[IBIS Ver]   4.1
[File Name]   tms570ls31x_21x_revb_pge_a.ibs
[File Rev]   1.0
[Date]   Tue Sep 17 07:21:23 2013
[Source]   Texas Instruments, Inc.
[Notes]   Revision History:
   1.0: initial release, 09/17/2013
   THIS IS RELEASE 1.0,THE CONTENTS ARE SUBJECT TO
   CHANGE WITHOUT PRIOR NOTICE,IF NECESSARY.
[Disclaimer] Please be aware that in the absence of a written agreement
   Texas Instruments(TI) assumes no liability for:
   (1) The accuracy of the IBIS models provided to your company
   (2) The proper functioning of these Models in your design
   or for any resulting applications;or
   (3) Infringement of patents,copyrights or intellectual
   property rights resulting from your use of these models.
   TI provides IBIS Models as a service to our customers and
   therefore reserves the right to limit distribution of the
   Models.
[Copyright]   Property of Texas Instruments Incorporated.
   Unauthorised reproduction and/or distribution is strictly.
   prohibited.
   This product is protected under copyright law and trade
   secret law as an unpublished work.
   Created 2013,(C) Copyright 2013-2014,
   Texas Instruments Incorporated., All Rights Reserved.
   These commodities are under the U.S. Government
   distribution license control.As such,they are not to be
   re-exported without the prior approval of the
   U.S. Department of Commerce.
[Component]   TMS570LS31x/21x_REVB_PGE_A
[Manufacturer]   Texas Instruments
[Package]
| variable   typ   min   max
R_pkg   203.864m   14.6492m   240.64m
L_pkg   7.02358nH   2.16743nH   7.77511nH
C_pkg   0.954257pF   0.768716pF   6.71726pF
[Pin]	signal_name	model_name	R_pin	L_pin	C_pin
1	GIOB[3]	BQ0210FT	222.975m	6.99501nH	0.93522pF
2	GIOA[0]	BQ0210FT	224.24m	7.38373nH	1.04917pF
3	MIBSPI3NCS[3]	BQ0210FT	223.892m	7.5187nH	1.04438pF
4	MIBSPI3NCS[2]	BQ0210FT	218.592m	7.59933nH	1.02569pF
5	GIOA[1]	BQ0210FT	218.18m	7.74551nH	1.00793pF
6	NHET1[11]	BQ0210FT	219.431m	7.77511nH	0.979037pF
|7	FLTP1	BAFTHRU15VFT	219.36m	7.69214nH	0.954057pF
|8	FLTP2	BAFTHRU8VFT	219.133m	7.68768nH	0.936523pF
9	GIOA[2]	BQ0215FT	222.776m	7.74151nH	0.909504pF
|10	VCCIO	VDDS33TF1_60UM	225.672m	7.66706nH	0.910106pF
|11	VSS	VSS00T2_60UM	224.592m	7.55399nH	0.899234pF
12	CAN3RX	BQ0210FT	225.127m	7.44625nH	0.865528pF
13	CAN3TX	BQ0210FT	233.703m	7.53614nH	0.859082pF
14	GIOA[5]	BQ0210FT	233.974m	7.45808nH	0.855654pF
15	NHET1[22]	BQ0215FT	234.031m	7.40297nH	0.854333pF
16	GIOA[6]	BQ0210FT	233.473m	7.31284nH	0.840194pF
|17	VCC	VDD12T1_100UM	143.652m	6.76561nH	0.863346pF
|18	OSCIN	IOSCHF33FTHY_NI	236.172m	7.35407nH	0.808573pF
|19	KELVIN_GND	VSS00T2_60UM	234.204m	7.32997nH	0.824803pF
|20	OSCOUT	OOSCHF33FT	230.471m	7.21233nH	0.834372pF
|21	VSS	VSS00T2_60UM	230.586m	7.16874nH	0.824864pF
22	GIOA[7]	BQ0210FT	229.213m	7.20298nH	0.824815pF
23	NHET1[01]	BQ0215FT	228.006m	7.16514nH	0.860924pF
24	NHET1[03]	BQ0215FT	227.34m	7.17463nH	0.878282pF
25	NHET1[0]	BQ0215FT	228.05m	7.17956nH	0.888602pF
|26	VCCIO	VDDS33TF1_60UM	142.679m	6.74705nH	0.965478pF
|27	VSS	VSS00T2_60UM	226.431m	7.1827nH	0.927108pF
|28	VSS	VSS00T2_60UM	226.676m	7.26977nH	0.947242pF
|29	VCC	VDD12T1_100UM	144.773m	6.89389nH	1.01996pF
30	NHET1[02]	BQ0215FT	224.882m	7.39158nH	0.965642pF
31	NHET1[05]	BQ0215FT	224.815m	7.46872nH	0.970215pF
32	MIBSPI5NCS[0]	BQ0210FT	224.229m	7.54786nH	1.00261pF
33	NHET1[07]	BQ0215FT	225.045m	7.61055nH	1.02855pF
34	TEST	BQ0213FT	230.338m	7.61528nH	1.04296pF
35	NHET1[09]	BQ0215FT	226.956m	7.38938nH	1.04678pF
36	NHET1[04]	BQ0210FT	224.889m	7.05005nH	0.930999pF
37	MIBSPI3NCS[1]	BQ0215FT	212.649m	6.95179nH	0.940286pF
38	NHET1[06]	BQ0210FT	209.151m	7.19337nH	1.05396pF
39	NHET1[13]	BQ0210FT	211.994m	7.38781nH	1.03563pF
40	MIBSPI1NCS[2]	BQ0215FT	203.865m	7.31168nH	1.02434pF
41	NHET1[15]	BQ0210FT	197.232m	7.17257nH	0.997865pF
|42	VCCIO	VDDS33TF1_60UM	193.515m	7.14097nH	0.960455pF
|43	VSS	VSS00T2_60UM	189.265m	7.01956nH	0.944505pF
|44	VSS	VSS00T2_60UM	187.979m	6.89986nH	0.934945pF
|45	VCC	VDD12T1_100UM	101.964m	6.14255nH	0.970118pF
46	nPORRST	IQ0087FT	188.154m	6.76798nH	0.87611pF
|47	VSS	VSS00T2_60UM	189.169m	6.716nH	0.871341pF
|48	VCC	VDD12T1_100UM	124.671m	6.12514nH	0.899774pF
|49	VCC	VDD12T1_100UM	124.517m	6.02737nH	0.884127pF
|50	VSS	VSS00T2_60UM	192.682m	6.41208nH	0.826834pF
51	MIBSPI3SOMI	BQ0211FT	190.675m	6.39926nH	0.804598pF
52	MIBSPI3SIMO	BQ0211FT	189.543m	6.38502nH	0.794641pF
53	MIBSPI3CLK	BQ0211FT	191.031m	6.44993nH	0.78565pF
54	MIBSPI3NENA	BQ0210FT	193.5m	6.48248nH	0.784395pF
55	MIBSPI3NCS[0]	BQ0210FT	196.751m	6.3841nH	0.784861pF
|56	VSS	VSS00T2_60UM	197.376m	6.37405nH	0.784546pF
|57	VCC	VDD12T1_100UM	99.2024m	5.75114nH	0.844285pF
|58	AD1IN[16]_AD2IN[0]	IQ0444FT5	187.646m	6.39966nH	0.792979pF
|59	AD1IN[17]_AD2IN[01]	IQ0444FT5	185.5m	6.52224nH	0.81771pF
|60	AD1IN[0]	IQ0078FT5	183.029m	6.49023nH	0.835845pF
|61	AD1IN[07]	IQ0078FT5	183.285m	6.51506nH	0.852657pF
|62	AD1IN[18]_AD2IN[02]	IQ0444FT5	182.225m	6.457nH	0.861357pF
|63	AD1IN[19]_AD2IN[03]	IQ0444FT5	180.283m	6.49189nH	0.869921pF
|64	AD1IN[20]_AD2IN[04]	IQ0444FT5	181.999m	6.61141nH	0.897543pF
|65	AD1IN[21]_AD2IN[05]	IQ0444FT5	183.721m	6.75667nH	0.916893pF
|66	ADREFHI	BAFTHRU50FT	184.523m	6.83056nH	0.928543pF
|67	ADREFLO	BAFTHRU50FT	188.003m	7.02503nH	0.948176pF
|68	VSSAD	VSSA00T2_100UM	190.277m	7.09058nH	0.985675pF
|69	VCCAD	VDDA50TF2	195.98m	7.15643nH	1.00819pF
|70	AD1IN[09]_AD2IN[09]	IQ0444FT5	201.155m	7.25699nH	1.03149pF
|71	AD1IN[01]	IQ0078FT5	206.74m	7.17571nH	1.05429pF
|72	AD1IN[10]_AD2IN[10]	IQ0444FT5	211.214m	6.94468nH	0.929652pF
|73	AD1IN[02]	IQ0078FT5	220.602m	7.13326nH	0.935756pF
|74	AD1IN[03]	IQ0078FT5	221.564m	7.53173nH	1.05755pF
|75	AD1IN[11]_AD2IN[11]	IQ0444FT5	220.565m	7.6612nH	1.03969pF
|76	AD1IN[04]	IQ0078FT5	218.103m	7.69725nH	1.02287pF
|77	AD1IN[12]_AD2IN[12]	IQ0444FT5	217.217m	7.7022nH	1.00582pF
|78	AD1IN[05]	IQ0078FT5	220.259m	7.69378nH	0.977311pF
|79	AD1IN[13]_AD2IN[13]	IQ0444FT5	220.272m	7.61159nH	0.965456pF
|80	AD1IN[06]	IQ0078FT5	221.46m	7.58304nH	0.955543pF
|81	AD1IN[22]_AD2IN[06]	IQ0444FT5	222.964m	7.59921nH	0.927212pF
|82	AD1IN[14]_AD2IN[14]	IQ0444FT5	223.626m	7.54273nH	0.902867pF
|83	AD1IN[08]_AD2IN[08]	IQ0444FT5	226.45m	7.46033nH	0.89311pF
|84	AD1IN[23]_AD2IN[07]	IQ0444FT5	229.464m	7.42855nH	0.881122pF
|85	AD1IN[15]_AD2IN[15]	IQ0444FT5	230.028m	7.31981nH	0.862162pF
86	AD1EVT	BQ0210FT	230.628m	7.23404nH	0.836966pF
|87	VCC	VDD12T1_100UM	115.681m	6.31505nH	0.922374pF
|88	VSS	VSS00T2_60UM	235.142m	7.02615nH	0.843683pF
89	CAN1TX	BQ0210FT	232.75m	7.08264nH	0.834243pF
90	CAN1RX	BQ0210FT	233.054m	7.11231nH	0.825741pF
91	NHET1[24]	BQ0210FT	234.357m	7.20193nH	0.824965pF
92	NHET1[26]	BQ0210FT	236.214m	7.26025nH	0.841317pF
93	MIBSPI1SIMO	BQ0211FT	238.667m	7.3379nH	0.841276pF
94	MIBSPI1SOMI	BQ0211FT	237.611m	7.33229nH	0.837111pF
95	MIBSPI1CLK	BQ0211FT	238.531m	7.37903nH	0.868579pF
96	MIBSPI1NENA	BQ0210FT	240.64m	7.43203nH	0.882242pF
97	MIBSPI5NENA	BQ0210FT	234.256m	7.3995nH	0.869613pF
98	MIBSPI5SOMI[0]	BQ0212FT	231.869m	7.37945nH	0.884338pF
99	MIBSPI5SIMO[0]	BQ0212FT	230.968m	7.43996nH	0.903187pF
100	MIBSPI5CLK	BQ0212FT	232.568m	7.51752nH	0.926711pF
|101	VCC	VDD12T1_100UM	226.934m	7.45028nH	0.937886pF
|102	VSS	VSS00T2_60UM	226.19m	7.4917nH	0.947092pF
|103	VSS	VSS00T2_60UM	224.556m	7.56386nH	0.973067pF
|104	VCCIO	VDDS33TF1_60UM	224.94m	7.58908nH	1.00754pF
105	MIBSPI1NCS[0]	BQ0215FT	222.915m	7.56045nH	1.02321pF
106	NHET1[08]	BQ0215FT	224.448m	7.58219nH	1.04229pF
107	NHET1[28]	BQ0215FT	222.931m	7.42217nH	1.04558pF
108	TMS	BQ0192FT	220.886m	7.05525nH	0.924796pF
109	nTRST	IQ0087FT	211.798m	7.03776nH	0.941307pF
110	TDI	BQ0192FT	207.154m	7.20508nH	1.06677pF
111	TDO	BQ0192FT	202.19m	7.26911nH	1.04213pF
112	TCK	IQ0079FT	194.436m	7.19682nH	1.00817pF
113	RTCK	OQ0112FT	192.036m	7.21931nH	0.967674pF
|114	VCC	VDD12T1_100UM	211.71m	7.51242nH	0.961463pF
|115	VSS	VSS00T2_60UM	203.678m	7.33374nH	0.951192pF
116	nRST	BQ0414FT	200.566m	7.26021nH	0.937088pF
117	nERROR	BQ0212FT	198.362m	7.0913nH	0.910275pF
118	NHET1[10]	BQ0215FT	199.266m	7.0054nH	0.890531pF
119	ECLK	BQ0215FT	196.87m	6.88885nH	0.87677pF
|120	VCCIO	VDDS33TF1_60UM	196.093m	6.64399nH	0.863029pF
|121	VSS	VSS00T2_60UM	189.351m	6.44196nH	0.839996pF
|122	VSS	VSS00T2_60UM	192.678m	6.39331nH	0.819925pF
|123	VCC	VDD12T1_100UM	124.076m	6.02398nH	0.843625pF
124	NHET1[12]	BQ0210FT	197.746m	6.48182nH	0.789005pF
125	NHET1[14]	BQ0215FT	195.58m	6.50716nH	0.777552pF
126	GIOB[0]	BQ0215FT	196.929m	6.5695nH	0.768716pF
127	NHET1[30]	BQ0215FT	194.122m	6.39736nH	0.774576pF
128	CAN2TX	BQ0210FT	191.055m	6.35392nH	0.77235pF
129	CAN2RX	BQ0210FT	194.643m	6.3988nH	0.799817pF
130	MIBSPI1NCS[1]	BQ0215FT	191.102m	6.35865nH	0.814533pF
131	LINRX	BQ0210FT	190.025m	6.39456nH	0.825368pF
132	LINTX	BQ0210FT	188.467m	6.4276nH	0.838409pF
133	GIOB[1]	BQ0215FT	186.875m	6.38656nH	0.841356pF
|134	VCCP	VDDFT33TF	121.74m	6.03022nH	0.892785pF
|135	VSS	VSS00T2_60UM	184.623m	6.49355nH	0.877041pF
|136	VCCIO	VDDS33TF1_60UM	183.838m	6.5272nH	0.907178pF
|137	VCC	VDD12T1_100UM	184.971m	6.68276nH	0.926105pF
|138	VSS	VSS00T2_60UM	185.732m	6.80371nH	0.937772pF
139	NHET1[16]	BQ0210FT	189.383m	6.91761nH	0.957847pF
140	NHET1[18]	BQ0210FT	193.514m	7.0503nH	0.994001pF
141	NHET1[20]	BQ0210FT	199.263m	7.13231nH	1.01201pF
142	GIOB[2]	BQ0210FT	204.28m	7.18696nH	1.03247pF
|143	VCC	VDD12T1_100UM	209.491m	7.13697nH	1.06099pF
|144	VSS	VSS00T2_60UM	213.612m	6.90639nH	0.943929pF
[Model Selector] BQ0192FT
BQ0192FT_PZ_3P3  Cell operated at 3.3(nom)
|BQ0192FT_PZ_3P3; PUPD_OFF
BQ0192FT_PU_3P3  Cell operated at 3.3(nom)
|BQ0192FT_PU_3P3; PULLUP_ON
BQ0192FT_PD_3P3  Cell operated at 3.3(nom)
|BQ0192FT_PD_3P3; PULLDOWN_ON
[Model Selector] BQ0210FT
BQ0210FT_PZ_3P3  Cell operated at 3.3(nom)
|BQ0210FT_PZ_3P3; PUPD_OFF
BQ0210FT_PU_3P3  Cell operated at 3.3(nom)
|BQ0210FT_PU_3P3; PULLUP_ON
BQ0210FT_PD_3P3  Cell operated at 3.3(nom)
|BQ0210FT_PD_3P3; PULLDOWN_ON
[Model Selector] BQ0211FT
BQ0211FT_PZ_3P3  Cell operated at 3.3(nom)
|BQ0211FT_PZ_3P3; PUPD_OFF
BQ0211FT_PU_3P3  Cell operated at 3.3(nom)
|BQ0211FT_PU_3P3; PULLUP_ON
BQ0211FT_PD_3P3  Cell operated at 3.3(nom)
|BQ0211FT_PD_3P3; PULLDOWN_ON
[Model Selector] BQ0212FT
BQ0212FT_PZ_3P3  Cell operated at 3.3(nom)
|BQ0212FT_PZ_3P3; PUPD_OFF
BQ0212FT_PU_3P3  Cell operated at 3.3(nom)
|BQ0212FT_PU_3P3; PULLUP_ON
BQ0212FT_PD_3P3  Cell operated at 3.3(nom)
|BQ0212FT_PD_3P3; PULLDOWN_ON
[Model Selector] BQ0213FT
BQ0213FT_PZ_3P3  Cell operated at 3.3(nom)
|BQ0213FT_PZ_3P3; PULLDOWN_OFF
BQ0213FT_PD_3P3  Cell operated at 3.3(nom)
|BQ0213FT_PD_3P3; PULLDOWN_ON
[Model Selector] BQ0215FT
BQ0215FT_PZ_3P3  Cell operated at 3.3(nom)
|BQ0215FT_PZ_3P3; PUPD_OFF
BQ0215FT_PU_3P3  Cell operated at 3.3(nom)
|BQ0215FT_PU_3P3; PULLUP_ON
BQ0215FT_PD_3P3  Cell operated at 3.3(nom)
|BQ0215FT_PD_3P3; PULLDOWN_ON
[Model Selector] BQ0414FT
BQ0414FT_PZ_3P3  Cell operated at 3.3(nom)
|BQ0414FT_PZ_3P3; PUPD_OFF
BQ0414FT_PU_3P3  Cell operated at 3.3(nom)
|BQ0414FT_PU_3P3; PULLUP_ON
BQ0414FT_PD_3P3  Cell operated at 3.3(nom)
|BQ0414FT_PD_3P3; PULLDOWN_ON
[Model Selector] IQ0079FT
IQ0079FT_PZ_3P3  Cell operated at 3.3(nom)
|IQ0079FT_PZ_3P3; PUPD_OFF
IQ0079FT_PU_3P3  Cell operated at 3.3(nom)
|IQ0079FT_PU_3P3; PULLUP_ON
IQ0079FT_PD_3P3  Cell operated at 3.3(nom)
|IQ0079FT_PD_3P3; PULLDOWN_ON
[Model Selector] IQ0087FT
IQ0087FT_PZ_3P3  Cell operated at 3.3(nom)
|IQ0087FT_PZ_3P3; PULLDOWN_OFF
IQ0087FT_PD_3P3  Cell operated at 3.3(nom)
|IQ0087FT_PD_3P3; PULLDOWN_ON
[Model Selector] IQ0442FT_40P60P
0442FT_40P60P_PZ_3P3  Cell operated at 3.3(nom)
|IQ0442FT_40P60P_PZ_3P3; PUPD_OFF
2FT_40P60P_PU_3P3  Cell operated at 3.3(nom)
|IQ0442FT_40P60P_PU_3P3; PULLUP_ON
2FT_40P60P_PD_3P3  Cell operated at 3.3(nom)
| Models and submodels in the file (29): BQ0192FT_PZ_3P3 (I/O), BQ0192FT_PU_3P3 (I/O), BQ0192FT_PD_3P3 (I/O), BQ0210FT_PZ_3P3 (I/O), BQ0210FT_PU_3P3 (I/O), BQ0210FT_PD_3P3 (I/O), BQ0211FT_PZ_3P3 (I/O), BQ0211FT_PU_3P3 (I/O), BQ0211FT_PD_3P3 (I/O), BQ0212FT_PZ_3P3 (I/O), BQ0212FT_PU_3P3 (I/O), BQ0212FT_PD_3P3 (I/O), BQ0213FT_PZ_3P3 (I/O), BQ0213FT_PD_3P3 (I/O), BQ0215FT_PZ_3P3 (I/O), BQ0215FT_PU_3P3 (I/O), BQ0215FT_PD_3P3 (I/O), BQ0414FT_PZ_3P3 (I/O), BQ0414FT_PU_3P3 (I/O), BQ0414FT_PD_3P3 (I/O), IQ0079FT_PZ_3P3 (Input), IQ0079FT_PU_3P3 (Input), IQ0079FT_PD_3P3 (Input), IQ0087FT_PZ_3P3 (Input), IQ0087FT_PD_3P3 (Input), 0442FT_40P60P_PZ_3P3 (Input), 2FT_40P60P_PU_3P3 (Input), 2FT_40P60P_PD_3P3 (Input), OQ0112FT (3-state)
